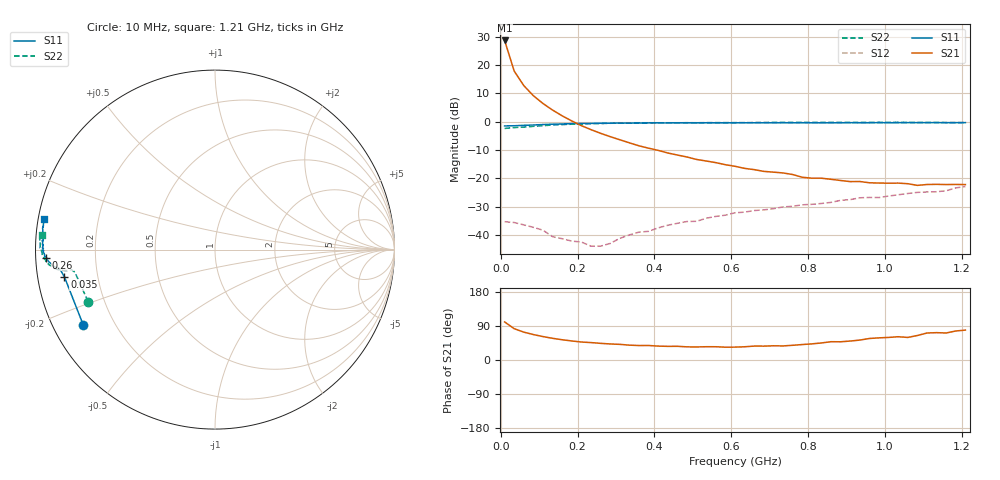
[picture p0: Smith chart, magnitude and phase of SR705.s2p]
!  POLYFET RF DEVICES
!  S PARAMETERS FOR
!  SR705 (EACH SIDE)
!  VDS=28, IDQ=600MA
! Date: Tue May 11 11:32:10 1999
# MHZ S MA R 50
! Freq=MHz Mag[s11] Ang[s11] Mag[s21] Ang[s21] Mag[s12] Ang[s12] Mag[s22] Ang[s22]
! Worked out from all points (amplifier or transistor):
!   49 points, 10 MHz to 1.21 GHz, reference 50 ohm
!   highest |S21| = 28.7 dB at 10 MHz (marker M1)
!   |S21| within 3 dB of that: start of sweep to 16.93 MHz
!   unconditionally stable (mu >= 1): 181.9 MHz to end of sweep
!   at 210 MHz: K = 1.12, MAG = 18.5 dB, |S12| = -42.4 dB
!   at 610 MHz: K = 1.26, MAG = 5.2 dB, |S12| = -32.1 dB
!   at 1.21 GHz: K = 1.22, MAG = -2.5 dB, |S12| = -22.9 dB
!   S11 on the Smith chart (normalised r, x): 10 MHz: 0.09, -0.26; 35 MHz: 0.08, -0.09; 260 MHz: 0.03, -0.02; 1.21 GHz: 0.02, +0.09
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10  0.8459 -150.1  27.27 100.4  0.01727 11.6  0.7639 -157.7
35  0.8524 -169.7  7.844 82.6  0.01668 -4.8  0.7909 -170.9
60  0.8667 -172.2  4.351 73.5  0.01517 -9.8  0.8074 -172.0
85  0.8776 -173.4  2.883 67.1  0.01372 -12.4  0.8323 -172.0
110  0.8957 -173.8  2.102 61.8  0.0122 -12.6  0.8551 -172.2
135  0.9075 -174.4  1.609 57.2  0.00938 -12.4  0.8785 -172.6
160  0.9159 -175.1  1.272 53.4  0.00864 -6.0  0.8932 -173.1
185  0.9276 -175.7  1.035 50.2  0.00784 14.1  0.9072 -173.6
210  0.935 -176.5  0.8546 47.5  0.00755 13.0  0.9115 -174.1
235  0.9374 -177.0  0.727 45.9  0.00638 31.5  0.9256 -174.6
260  0.9428 -177.3  0.6258 43.9  0.00638 44.5  0.9313 -175.1
335  0.9498 -178.2  0.4255 39.2  0.01008 71.4  0.9467 -176.6
385  0.9563 -179.2  0.3422 38.3  0.01165 85.0  0.9528 -177.3
410  0.9581 -179.5  0.313 36.7  0.01342 86.2  0.9555 -177.6
510  0.9559 179.6  0.2164 34.4  0.01753 92.5  0.962 -178.9
610  0.959 178.5  0.1639 34.0  0.02477 96.7  0.9674 -179.6
810  0.9604 177.1  0.1011 42.6  0.03493 105.3  0.9744 178.2
935  0.9636 175.0  0.0883 52.6  0.04556 106.1  0.9724 177.5
1010  0.9631 174.7  0.08243 59.6  0.04888 107.9  0.9785 176.7
1085  0.9665 172.3  0.07548 64.6  0.05677 107.0  0.9739 175.9
1160  0.9653 172.2  0.07806 71.3  0.06071 112.9  0.9696 175.3
1210  0.9689 169.9  0.07795 78.9  0.07199 108.9  0.9667 175.0
